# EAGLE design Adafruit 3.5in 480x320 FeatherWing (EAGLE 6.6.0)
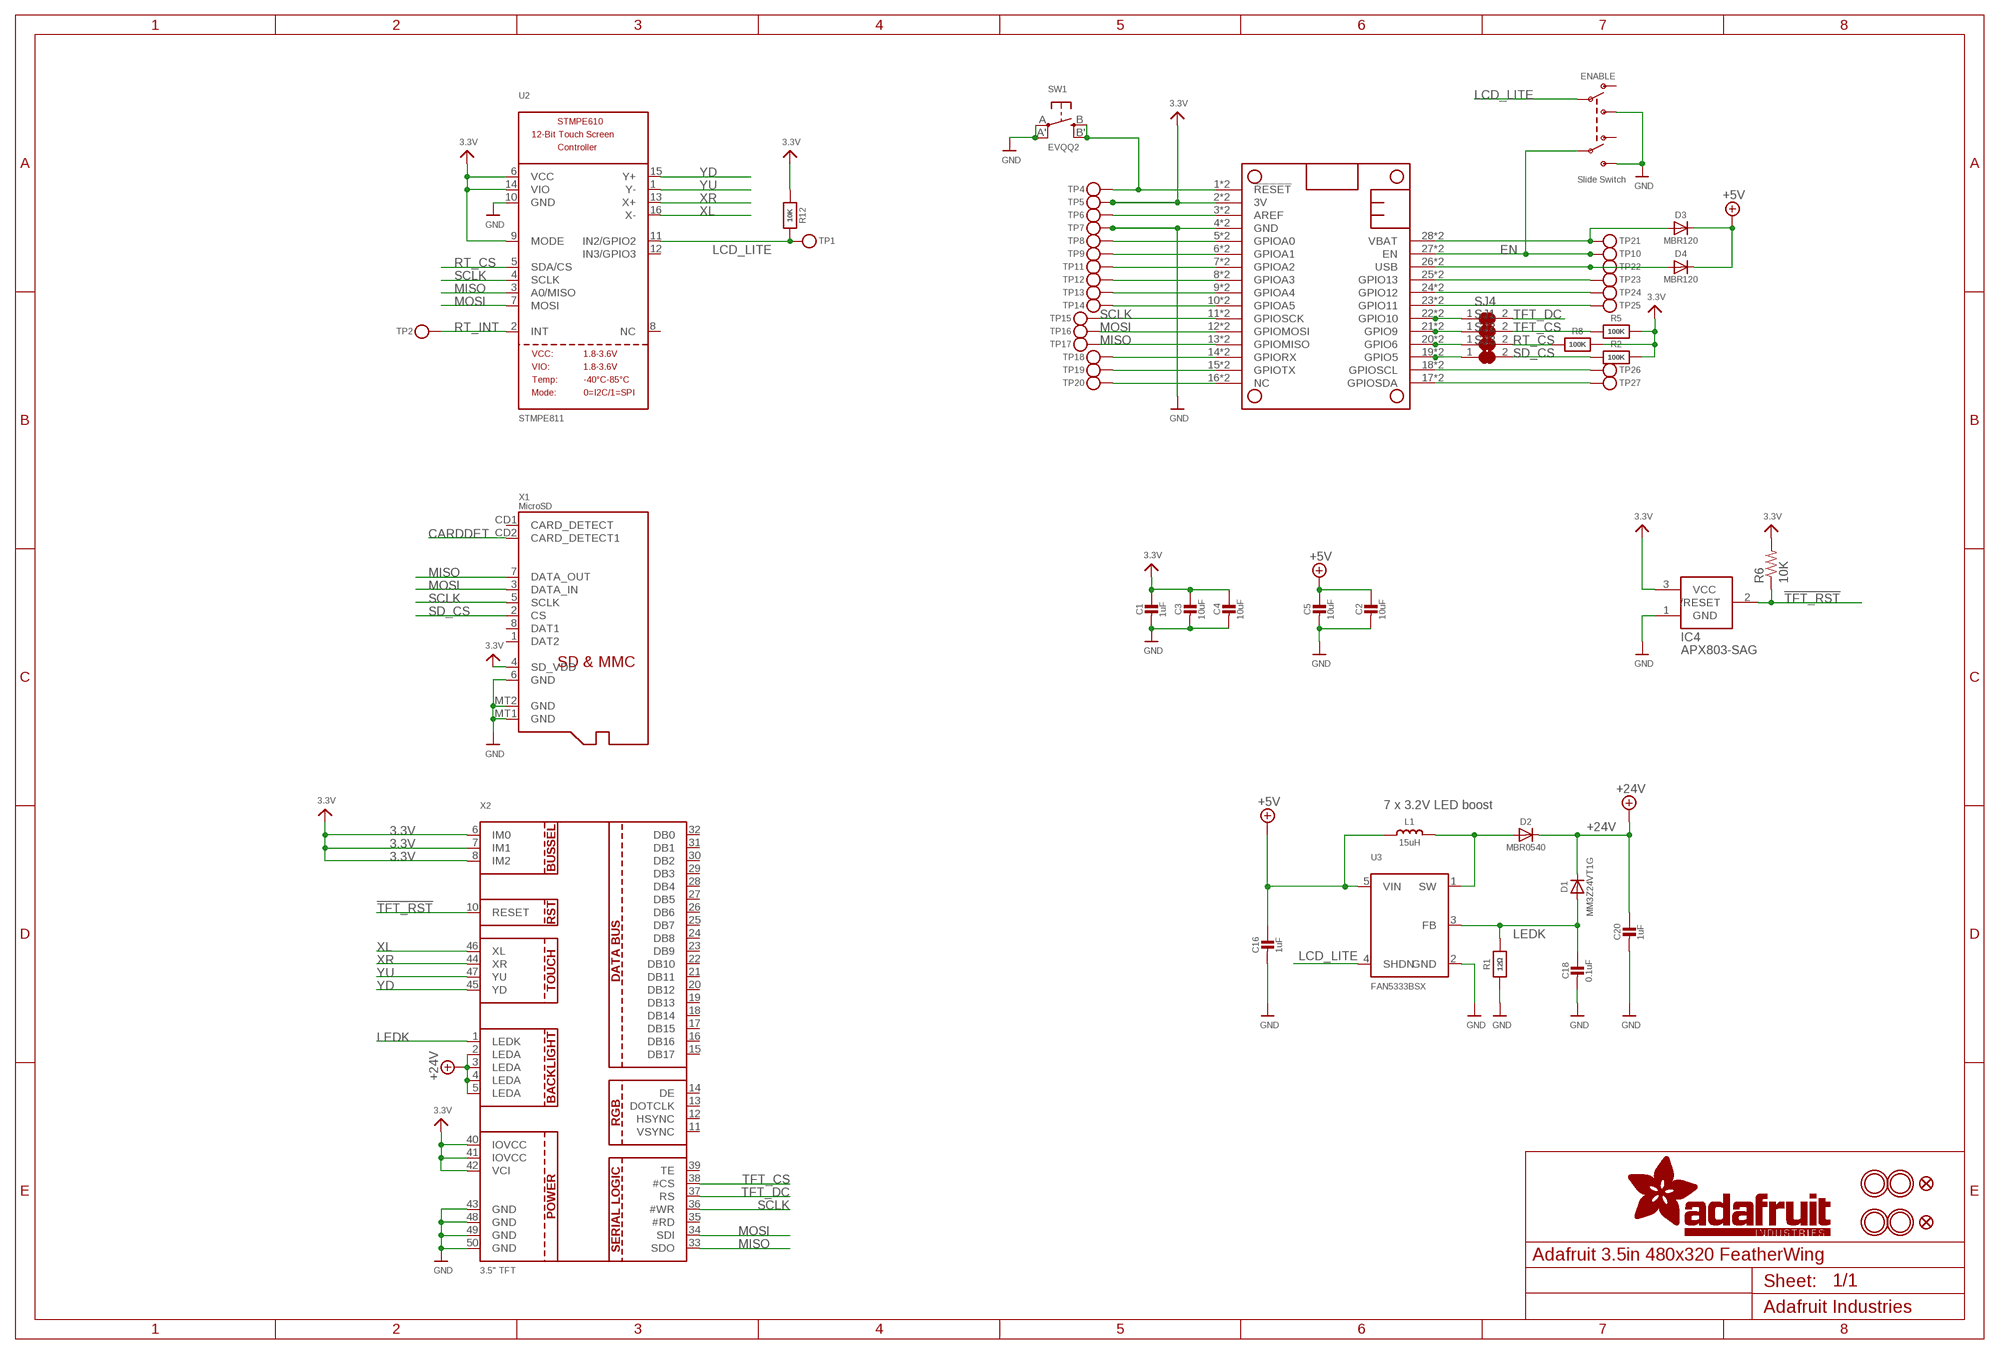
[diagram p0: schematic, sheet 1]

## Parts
C1  1uF  CAP_CERAMIC0805-NOOUTLINE  [0805-NO]
C2  10uF  CAP_CERAMIC0805-NOOUTLINE  [0805-NO]
C3  10uF  CAP_CERAMIC0805-NOOUTLINE  [0805-NO]
C4  10uF  CAP_CERAMIC0805-NOOUTLINE  [0805-NO]
C5  10uF  CAP_CERAMIC0805-NOOUTLINE  [0805-NO]
C16  1uF  CAP_CERAMIC0805-NOOUTLINE  [0805-NO]
C18  0.1uF  CAP_CERAMIC0805-NOOUTLINE  [0805-NO]
C20  1uF  CAP_CERAMIC0805-NOOUTLINE  [0805-NO]
D1  MM3Z24VT1G  DIODESMA  [SMADIODE]
D2  MBR0540  DIODESOD-123  [SOD-123]
D3  MBR120  DIODESOD-123  [SOD-123]
D4  MBR120  DIODESOD-123  [SOD-123]
ENABLE  Slide Switch  SWITCH_DPDTEG1390  [EG1390]
IC4  APX803-SAG  AXP083-SAG  [SOT23]
L1  15uH  INDUCTORNR5040  [INDUCTOR_5X5MM_NR5040_NOTHERMALS]
MS2  FEATHERWING_SMTDUAL  [FEATHERWING_SMT2]
R1  12Ω  RESISTOR0805_NOOUTLINE  [0805-NO]
R2  100K  RESISTOR0805_NOOUTLINE  [0805-NO]
R5  100K  RESISTOR0805_NOOUTLINE  [0805-NO]
R6  10K  R-US_R0805  [R0805]
R8  100K  RESISTOR0805_NOOUTLINE  [0805-NO]
R12  10K  RESISTOR0805_NOOUTLINE  [0805-NO]
SJ1  SOLDERJUMPER_CLOSED  [SOLDERJUMPER_CLOSEDWIRE]
SJ2  SOLDERJUMPER_CLOSED  [SOLDERJUMPER_CLOSEDWIRE]
SJ3  SOLDERJUMPER_CLOSED  [SOLDERJUMPER_CLOSEDWIRE]
SJ4  SOLDERJUMPER_CLOSED  [SOLDERJUMPER_CLOSEDWIRE]
SW1  EVQQ2  SWITCH_TACT_SMT_EVQQ2_SMALL  [EVQ-Q2_SMALLER]
TP1  TESTPOINTPAD2MM  [TESTPOINT_PAD_2MM]
TP2  TESTPOINTPAD2MM  [TESTPOINT_PAD_2MM]
TP4  TESTPOINTPAD2MM  [TESTPOINT_PAD_2MM]
TP5  TESTPOINTPAD2MM  [TESTPOINT_PAD_2MM]
TP6  TESTPOINTPAD2MM  [TESTPOINT_PAD_2MM]
TP7  TESTPOINTPAD2MM  [TESTPOINT_PAD_2MM]
TP8  TESTPOINTPAD2MM  [TESTPOINT_PAD_2MM]
TP9  TESTPOINTPAD2MM  [TESTPOINT_PAD_2MM]
TP10  TESTPOINTPAD2MM  [TESTPOINT_PAD_2MM]
TP11  TESTPOINTPAD2MM  [TESTPOINT_PAD_2MM]
TP12  TESTPOINTPAD2MM  [TESTPOINT_PAD_2MM]
TP13  TESTPOINTPAD2MM  [TESTPOINT_PAD_2MM]
TP14  TESTPOINTPAD2MM  [TESTPOINT_PAD_2MM]
TP15  TESTPOINTPAD2MM  [TESTPOINT_PAD_2MM]
TP16  TESTPOINTPAD2MM  [TESTPOINT_PAD_2MM]
TP17  TESTPOINTPAD2MM  [TESTPOINT_PAD_2MM]
TP18  TESTPOINTPAD2MM  [TESTPOINT_PAD_2MM]
TP19  TESTPOINTPAD2MM  [TESTPOINT_PAD_2MM]
TP20  TESTPOINTPAD2MM  [TESTPOINT_PAD_2MM]
TP21  TESTPOINTPAD2MM  [TESTPOINT_PAD_2MM]
TP22  TESTPOINTPAD2MM  [TESTPOINT_PAD_2MM]
TP23  TESTPOINTPAD2MM  [TESTPOINT_PAD_2MM]
TP24  TESTPOINTPAD2MM  [TESTPOINT_PAD_2MM]
TP25  TESTPOINTPAD2MM  [TESTPOINT_PAD_2MM]
TP26  TESTPOINTPAD2MM  [TESTPOINT_PAD_2MM]
TP27  TESTPOINTPAD2MM  [TESTPOINT_PAD_2MM]
U2  STMPE811  STMPE610  [QFN16_3MM]
U3  FAN5333BSX  FAN5331  [SOT23-5@1]
U$7  MOUNTINGHOLE3.0THIN  [MOUNTINGHOLE_3.0_PLATEDTHIN]
U$9  FIDUCIAL_1MM  [FIDUCIAL_1MM]
U$15  MOUNTINGHOLE3.0THIN  [MOUNTINGHOLE_3.0_PLATEDTHIN]
U$16  MOUNTINGHOLE3.0THIN  [MOUNTINGHOLE_3.0_PLATEDTHIN]
U$17  MOUNTINGHOLE3.0THIN  [MOUNTINGHOLE_3.0_PLATEDTHIN]
U$23  FIDUCIAL_1MM  [FIDUCIAL_1MM]
X1  MicroSD  MICROSD  [MICROSD]
X2  3.5" TFT  DISP_LCD_3.5IN_320X480_50PIN  [TFT_3.5IN_320X480_50PIN]

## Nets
3.3V: C1.1 C3.1 C4.1 IC4.3(VCC) MS2.2'(3V) MS2.2(3V) R2.2 R5.2 R6.2 R8.2 R12.1 TP5.P$1 U2.6(VCC) U2.9(MODE) U2.14(VIO) X1.4(SD_VDD) X2.6(IM0) X2.7(IM1) X2.8(IM2) X2.40(IOVCC) X2.41(IOVCC) X2.42(VCI)
!RESET: MS2.1'(!RESET) MS2.1(!RESET) SW1.B'(S1) SW1.B(S) TP4.P$1
!TFT_RST: IC4.2(/RESET) R6.1 X2.10(RESET)
+5V: C2.1 C5.1 C16.1 D3.C D4.C L1.P$1 U3.5(VIN)
+24V: C20.1 D1.C D2.C X2.2(LEDA) X2.3(LEDA) X2.4(LEDA) X2.5(LEDA)
A: MS2.5'(GPIOA0) MS2.5(GPIOA0) TP8.P$1
AREF: MS2.3'(AREF) MS2.3(AREF) TP6.P$1
B: MS2.6'(GPIOA1) MS2.6(GPIOA1) TP9.P$1
C: MS2.7'(GPIOA2) MS2.7(GPIOA2) TP11.P$1
CARDDET: X1.CD2(CARD_DETECT1)
D: MS2.8'(GPIOA3) MS2.8(GPIOA3) TP12.P$1
E: MS2.9'(GPIOA4) MS2.9(GPIOA4) TP13.P$1
EN: ENABLE.P2 MS2.27'(EN) MS2.27(EN) TP10.P$1
F: MS2.10'(GPIOA5) MS2.10(GPIOA5) TP14.P$1
G: MS2.16'(NC) MS2.16(NC) TP20.P$1
GND: C1.2 C2.2 C3.2 C4.2 C5.2 C16.2 C18.2 C20.2 ENABLE.S1 ENABLE.S2 IC4.1(GND) MS2.4'(GND) MS2.4(GND) R1.1 SW1.A'(P1) SW1.A(P) TP7.P$1 U2.10(GND) U3.2(GND) X1.6(GND) X1.MT1(GND) X1.MT2(GND) X2.43(GND) X2.48(GND) X2.49(GND) X2.50(GND)
H: MS2.19'(GPIO5) MS2.19(GPIO5) SJ3.1
I: MS2.20'(GPIO6) MS2.20(GPIO6) SJ2.1
J: MS2.21'(GPIO9) MS2.21(GPIO9) SJ1.1
K: MS2.22'(GPIO10) MS2.22(GPIO10) SJ4.1
L: MS2.23'(GPIO11) MS2.23(GPIO11) TP25.P$1
LCD_LITE: ENABLE.P1 R12.2 TP1.P$1 U2.11(IN2/GPIO2) U3.4(SHDN)
LEDK: C18.1 D1.A R1.2 U3.3(FB) X2.1(LEDK)
M: MS2.24'(GPIO12) MS2.24(GPIO12) TP24.P$1
MISO: MS2.13'(GPIOMISO) MS2.13(GPIOMISO) TP17.P$1 U2.3(A0/MISO) X1.7(DATA_OUT) X2.33(SDO)
MOSI: MS2.12'(GPIOMOSI) MS2.12(GPIOMOSI) TP16.P$1 U2.7(MOSI) X1.3(DATA_IN) X2.34(SDI)
N: MS2.25'(GPIO13) MS2.25(GPIO13) TP23.P$1
N$3: D2.A L1.P$2 U3.1(SW)
RT_CS: R8.1 SJ2.2 U2.5(SDA/CS)
RT_INT: TP2.P$1 U2.2(INT)
RX: MS2.14'(GPIORX) MS2.14(GPIORX) TP18.P$1
SCL: MS2.18'(GPIOSCL) MS2.18(GPIOSCL) TP26.P$1
SCLK: MS2.11'(GPIOSCK) MS2.11(GPIOSCK) TP15.P$1 U2.4(SCLK) X1.5(SCLK) X2.36(#WR)
SD_CS: R2.1 SJ3.2 X1.2(CS)
SDA: MS2.17'(GPIOSDA) MS2.17(GPIOSDA) TP27.P$1
TFT_CS: R5.1 SJ1.2 X2.38(#CS)
TFT_DC: SJ4.2 X2.37(RS)
TX: MS2.15'(GPIOTX) MS2.15(GPIOTX) TP19.P$1
USB: D4.A MS2.26'(USB) MS2.26(USB) TP22.P$1
VBAT: D3.A MS2.28'(VBAT) MS2.28(VBAT) TP21.P$1
XL: U2.16(X-) X2.46(XL)
XR: U2.13(X+) X2.44(XR)
YD: U2.15(Y+) X2.45(YD)
YU: U2.1(Y-) X2.47(YU)
Unconnected: ENABLE.O1 ENABLE.O2 U2.8(NC) U2.12(IN3/GPIO3) X1.1(DAT2) X1.8(DAT1) X1.CD1(CARD_DETECT) X2.11(VSYNC) X2.12(HSYNC) X2.13(DOTCLK) X2.14(DE) X2.15(DB17) X2.16(DB16) X2.17(DB15) X2.18(DB14) X2.19(DB13) X2.20(DB12) X2.21(DB11) X2.22(DB10) X2.23(DB9) X2.24(DB8) X2.25(DB7) X2.26(DB6) X2.27(DB5) X2.28(DB4) X2.29(DB3) X2.30(DB2) X2.31(DB1) X2.32(DB0) X2.35(#RD) X2.39(TE)

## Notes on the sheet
- 7 x 3.2V LED boost

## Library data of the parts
C1-C5 C16 C18 C20 = microbuilder:CAP_CERAMIC: Ceramic Capacitors
D1-D4 = microbuilder:DIODE: Diode
ENABLE = microbuilder:SWITCH_DPDT: Switch - DPDT A DPDT Switch acts like an SPDT switch, but has a pair of switches instead of just one. Vertical - 0.3A @ 6V SMT - Digikey: JS202011SCQN
IC4 = adafruit:AXP083
L1 = microbuilder:INDUCTOR: Inductors
MS2 = microbuilder:FEATHERWING
R1 R2 R5 R8 R12 = microbuilder:RESISTOR: Resistors
R6 = rcl:R-US_: RESISTOR, American symbol
SJ1-SJ4 = microbuilder:SOLDERJUMPER_CLOSED: Solder Jumper - Closed
SW1 = microbuilder:SWITCH_TACT_SMT: SMT Tact Switches 6x6mm - Digikey: P12940SCT-ND KMR2 (4.6x2.8mm) - Digikey: 401-1426-1-ND EVQ-PQHB55 - Light Touch, 160GF (4.5x4.5mm) - Digikey: P8090SCT-ND KMT0 - KMT021 NGJ LHS (etc.) IP68/Waterproof - Digikey: CKN10289CT-ND
TP1 TP2 TP4-TP27 = microbuilder:TESTPOINT: Test Point
U2 = microbuilder:STMPE610: STMPE610 - 12-Bit Touch Screen Controller
U3 = microbuilder:FAN5331: FAN5331 - LED/OLED 20V Boost Converter Digikey: FAN5331SXCT-ND
U$7 U$15-U$17 = microbuilder:MOUNTINGHOLE: Mounting Hole; BOM: EXCLUDE
U$9 U$23 = microbuilder:FIDUCIAL: Fiducial Alignment Points; BOM: EXCLUDE
X1 = microbuilder:MICROSD: MicroSD/Transflash Card Holder with SPI pinout 3M: 2908-05WB-MG 4UConnector: 19656 Footprint courtesy: Adafruit Industries
X2 = microbuilder:DISP_LCD_3.5IN_320X480_50PIN: DT350HV15-T - 3.5" 320x480 TFT Display, 50 Pin Connector

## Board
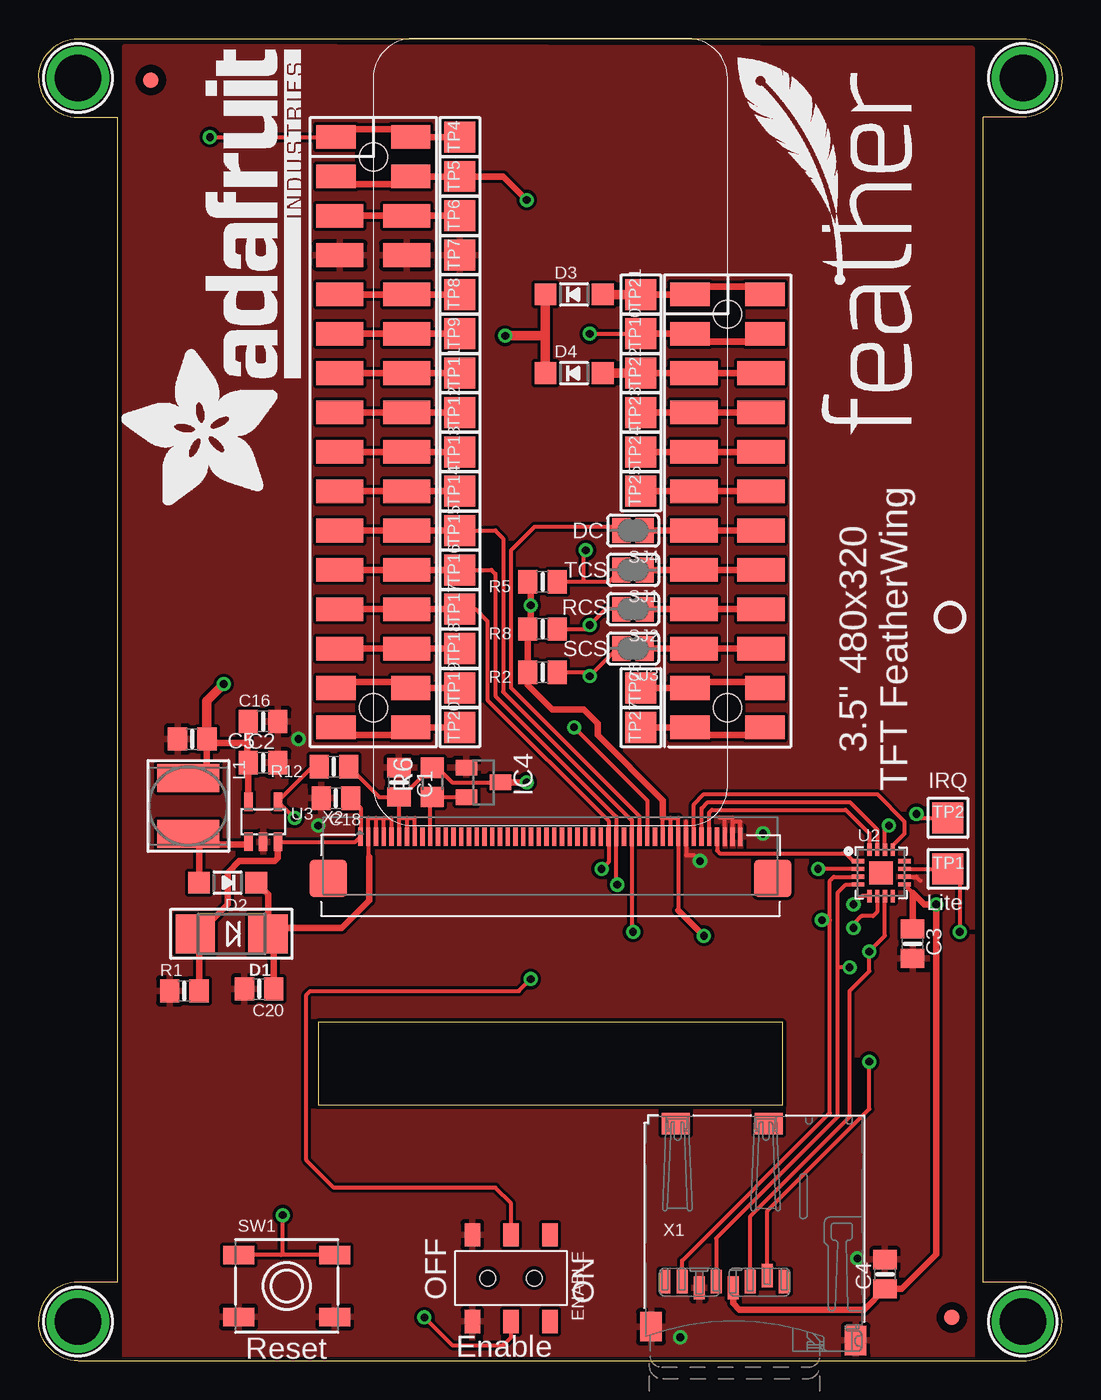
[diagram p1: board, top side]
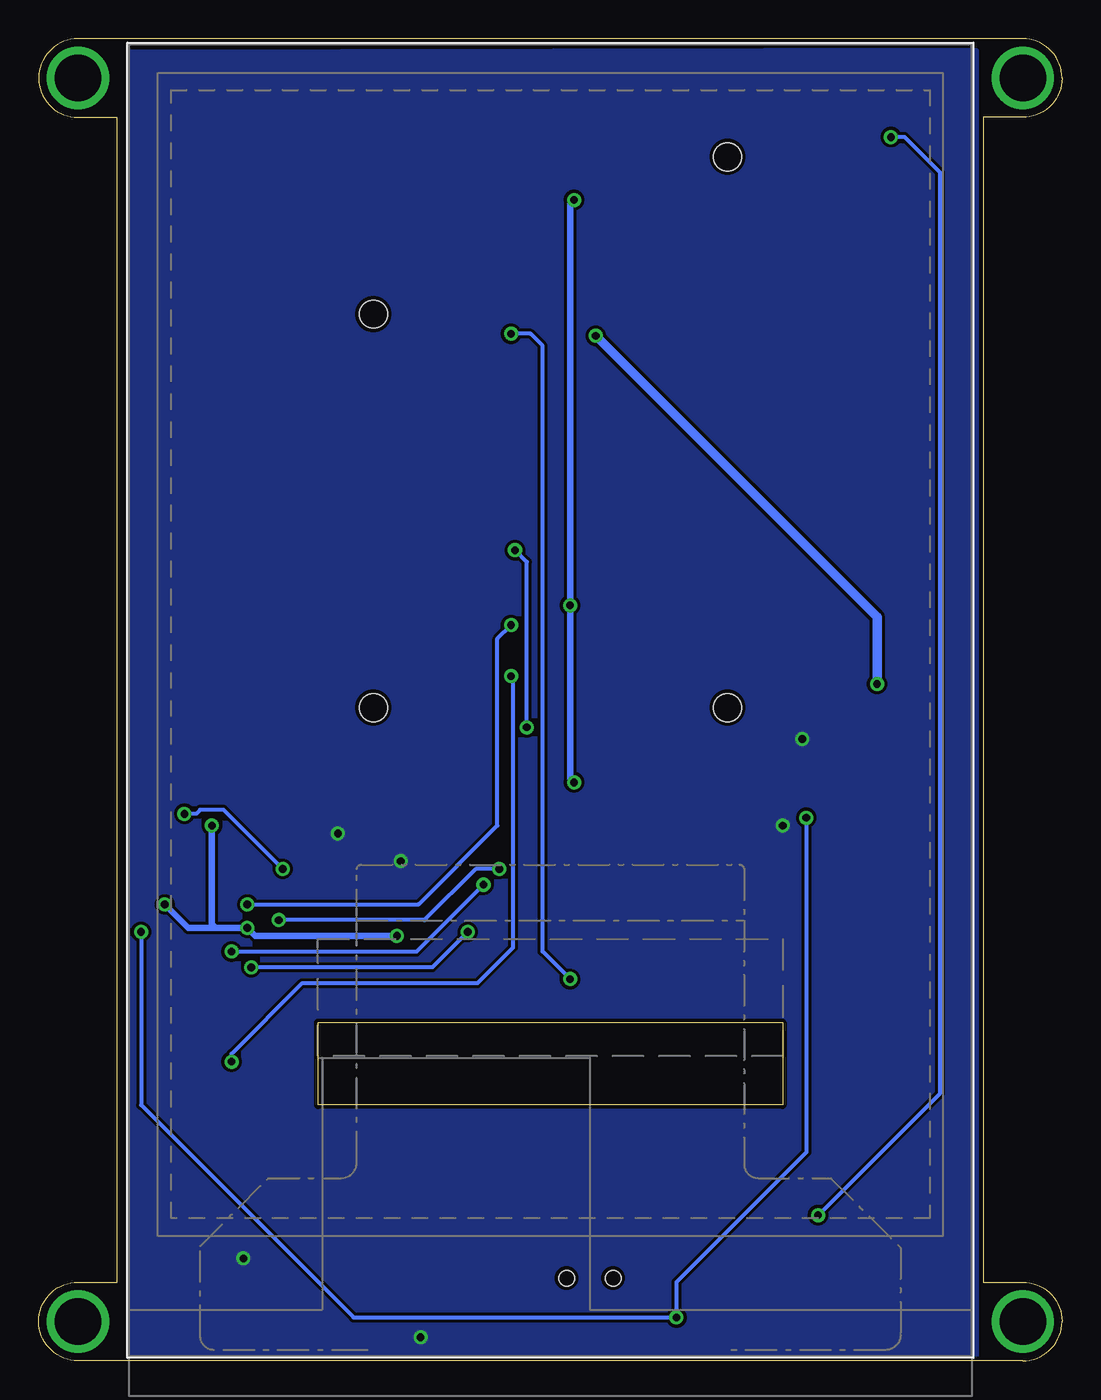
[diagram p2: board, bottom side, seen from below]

Size 66.04 x 85.34 mm. Coordinates in mm from the lower left corner, seen from the top.
Outline: 2.54,0 63.5,0 arc90 66.04,2.54 arc90 63.5,5.08 60.96,5.08 60.96,80.26 63.5,80.26 arc90 66.04,82.8 arc90 63.5,85.34 2.54,85.34 arc90 0,82.8 arc90 2.54,80.26 5.08,80.26 5.08,5.08 2.54,5.08 arc90 0,2.54 arc90 2.54,0
Outline: 18.03,21.84 18.03,16.51 48.01,16.51 48.01,21.84 18.03,21.84
Copper layers (1*16): Top 0.035mm / dielectric 1.5mm / Bottom 0.035mm
Design rules "adafruit *": minimum track width 8mil, minimum drill 15.5mil, track to track 8mil, track to pad 8mil, pad to pad 8mil, via to via 8mil, smd to smd 8mil, copper to edge 10mil, drill to drill 8mil, minimum pad ring 10mil, minimum via ring 8mil, stop-mask expansion 2mil, vias tented up to drill 20mil, thermal gap 10mil
tRestrict: area 44.5,33.7 to 44.6,34; area 45,33.7 to 45.1,34

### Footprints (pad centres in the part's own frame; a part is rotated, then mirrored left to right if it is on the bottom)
0805-NO = smd 1.24 x 1.5: 1 -0.95,0; 2 0.95,0
SMADIODE = smd 2.54 x 2.54: A 2.349,0; C -2.349,0
SOD-123 = smd 1.4 x 1.4: A 1.85,0; C -1.85,0
EG1390 = smd 1 x 1.5: O1 -2.5,2.8; O2 -2.5,-2.8; P1 0,2.8; P2 0,-2.8; S1 2.5,2.8; S2 2.5,-2.8 | hole 1: 1.5,0; -1.5,0
SOT23 = smd 1 x 1.4: 1 -0.95,-1.1; 2 0.95,-1.1; 3 0,1.1
INDUCTOR_5X5MM_NR5040_NOTHERMALS = smd 1.8 x 4: P$1 -1.8,0; P$2 1.8,0
FEATHERWING_SMT2 = smd 1.524 x 2.54: 1 6.35,2.413; 1' 6.35,-2.413; 2 8.89,2.413; 2' 8.89,-2.413; 15 41.91,2.413; 15' 41.91,-2.413; 16 44.45,2.413; 16' 44.45,-2.413; 17 44.45,20.447; 17' 44.45,25.273; 18 41.91,20.447; 18' 41.91,25.273; 27 19.05,20.447; 27' 19.05,25.273; 28 16.51,20.447; 28' 16.51,25.273 | smd 1.524 x 3.048: 3 11.43,2.159; 3' 11.43,-2.159; 4 13.97,2.159; 4' 13.97,-2.159; 5 16.51,2.159; 5' 16.51,-2.159; 6 19.05,2.159; 6' 19.05,-2.159; 7 21.59,2.159; 7' 21.59,-2.159; 8 24.13,2.159; 8' 24.13,-2.159; 9 26.67,2.159; 9' 26.67,-2.159; 10 29.21,2.159; 10' 29.21,-2.159; 11 31.75,2.159; 11' 31.75,-2.159; 12 34.29,2.159; 12' 34.29,-2.159; 13 36.83,2.159; 13' 36.83,-2.159; 14 39.37,2.159; 14' 39.37,-2.159; 19 39.37,20.701; 19' 39.37,25.019; 20 36.83,20.701; 20' 36.83,25.019; 21 34.29,20.701; 21' 34.29,25.019; 22 31.75,20.701; 22' 31.75,25.019; 23 29.21,20.701; 23' 29.21,25.019; 24 26.67,20.701; 24' 26.67,25.019; 25 24.13,20.701; 25' 24.13,25.019; 26 21.59,20.701; 26' 21.59,25.019 | hole 1.8: 17.78,22.86; 43.18,22.86; 7.62,0; 43.18,0
R0805 = smd 1.3 x 1.5: 1 -0.95,0; 2 0.95,0
SOLDERJUMPER_CLOSEDWIRE = smd 1.168 x 1.6: 1 -0.762,0; 2 0.762,0 | smd 0.635 x 0.203: WIRE 0,0
EVQ-Q2_SMALLER = smd 2 x 1.2: A -3.1,-2; A' 3.1,-2; B -3.1,2; B' 3.1,2
TESTPOINT_PAD_2MM = smd 2 x 2: P$1 0,0
QFN16_3MM = smd 0.8 x 0.28: 1 -1.5,0.75; 2 -1.5,0.25; 3 -1.5,-0.25; 4 -1.5,-0.75; 9 1.5,-0.75; 10 1.5,-0.25; 11 1.5,0.25; 12 1.5,0.75 | smd 0.28 x 0.8: 5 -0.75,-1.5; 6 -0.25,-1.5; 7 0.25,-1.5; 8 0.75,-1.5; 13 0.75,1.5; 14 0.25,1.5; 15 -0.25,1.5; 16 -0.75,1.5 | smd 1.5 x 1.5: THERMAL 0,0
SOT23-5@1 = smd 0.55 x 1.2: 1 -0.95,-1.3; 2 0,-1.3; 3 0.95,-1.3; 4 0.95,1.3; 5 -0.95,1.3
MOUNTINGHOLE_3.0_PLATEDTHIN = drill 3 pad 3.6: P$1 0,0
FIDUCIAL_1MM = smd 1 x 1: 1 0,0
MICROSD = smd 0.7 x 1.5: 1 9,-10.64; 2 7.9,-10.24; 3 6.8,-10.64; 4 5.7,-11.04; 5 4.6,-10.64; 6 3.5,-11.04; 7 2.4,-10.64; 8 1.3,-10.64 | smd 1.8 x 1.4: CD1 2,-0.44; CD2 8,-0.44 | smd 1.4 x 1.9: MT1 0.4,-13.54; MT2 13.6,-14.44
TFT_3.5IN_320X480_50PIN = smd 0.275 x 1.2 bottom: 1 12.25,-3.76; 2 11.75,-3.76; 3 11.25,-3.76; 4 10.75,-3.76; 5 10.25,-3.76; 6 9.75,-3.76; 7 9.25,-3.76; 8 8.75,-3.76; 9 8.25,-3.76; 10 7.75,-3.76; 11 7.25,-3.76; 12 6.75,-3.76; 13 6.25,-3.76; 14 5.75,-3.76; 15 5.25,-3.76; 16 4.75,-3.76; 17 4.25,-3.76; 18 3.75,-3.76; 19 3.25,-3.76; 20 2.75,-3.76; 21 2.25,-3.76; 22 1.75,-3.76; 23 1.25,-3.76; 24 0.75,-3.76; 25 0.25,-3.76; 26 -0.25,-3.76; 27 -0.75,-3.76; 28 -1.25,-3.76; 29 -1.75,-3.76; 30 -2.25,-3.76; 31 -2.75,-3.76; 32 -3.25,-3.76; 33 -3.75,-3.76; 34 -4.25,-3.76; 35 -4.75,-3.76; 36 -5.25,-3.76; 37 -5.75,-3.76; 38 -6.25,-3.76; 39 -6.75,-3.76; 40 -7.25,-3.76; 41 -7.75,-3.76; 42 -8.25,-3.76; 43 -8.75,-3.76; 44 -9.25,-3.76; 45 -9.75,-3.76; 46 -10.25,-3.76; 47 -10.75,-3.76; 48 -11.25,-3.76; 49 -11.75,-3.76; 50 -12.25,-3.76 | smd 2.4 x 2.4 bottom: PAD1 14.35,-6.46; PAD2 -14.35,-6.46

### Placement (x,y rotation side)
C1  23.24,37.34 90 top
C2  14.48,38.61 0 top
C3  56.39,26.92 270 top
C4  54.61,5.59 90 top
C5  9.91,40.13 180 top
C16  14.48,41.27 0 top
C18  19.18,36.32 180 top
C20  14.22,24 180 top
D1  12.45,27.56 180 top
D2  12.19,30.86 180 top
D3  34.54,68.83 0 top
D4  34.54,63.75 0 top
ENABLE  30.48,5.33 180 top
IC4  28.7,37.34 270 top
L1  9.65,35.81 270 top
MS2  21.59,85.34 270 top
R1  9.4,23.88 0 top
R2  32.51,44.45 180 top
R5  32.51,50.29 180 top
R6  25.4,37.34 90 top
R8  32.51,47.24 180 top
R12  19.05,38.35 180 top
SJ1  38.35,51.05 180 top
SJ2  38.35,48.51 180 top
SJ3  38.35,45.97 180 top
SJ4  38.35,53.59 180 top
SW1  16,4.83 0 top
TP1  58.67,31.75 0 top
TP2  58.67,35.05 0 top
TP4  27.18,78.99 90 top
TP5  27.18,76.45 90 top
TP6  27.18,73.91 90 top
TP7  27.18,71.37 90 top
TP8  27.18,68.83 90 top
TP9  27.18,66.29 90 top
TP10  38.86,66.29 90 top
TP11  27.18,63.75 90 top
TP12  27.18,61.21 90 top
TP13  27.18,58.67 90 top
TP14  27.18,56.13 90 top
TP15  27.18,53.59 90 top
TP16  27.18,51.05 90 top
TP17  27.18,48.51 90 top
TP18  27.18,45.97 90 top
TP19  27.18,43.43 90 top
TP20  27.18,40.89 90 top
TP21  38.86,68.83 90 top
TP22  38.86,63.75 90 top
TP23  38.86,61.21 90 top
TP24  38.86,58.67 90 top
TP25  38.86,56.13 90 top
TP26  38.86,43.43 90 top
TP27  38.86,40.89 90 top
U2  54.36,31.5 0 top
U3  14.48,34.8 0 top
U$7  2.54,2.54 0 top
U$9  58.93,2.79 0 top
U$11  [FEATHERLOGO]  56.39,59.82 90 top
U$15  63.5,2.54 0 top
U$16  2.54,82.8 0 top
U$17  63.5,82.8 0 top
U$19  [ADAFRUIT_TEXT_30MM]  16.89,54.99 90 top
U$23  7.24,82.68 0 top
U$37  [PCBFEAT-REV-040]  58.8,48.01 90 top
X1  39.12,15.75 0 top
X2  33.02,37.59 0 bottom

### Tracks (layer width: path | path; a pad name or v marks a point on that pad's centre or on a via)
3.3V  (via drill 0.5)
  Top 0.254: X2.6 23.27,35.05 | 23.27,35.05 23.77,35.05 | 23.77,35.05 24.27,35.05 X2.8 | X2.7 23.77,35.05 | 23.27,35.05 23.27,36.39 C1.1 | C1.1 23.43,36.39 24.89,37.85 24.96,37.85 R6.2 25.72,38.29 26.67,37.34 IC4.3 | U2.9 56.39,30.21 | U2.6 54.11,28.96 53.85,28.7 53.09,28.7 52.58,28.19 v52.58,27.94 | X2.40 40.27,35.05 40.77,35.05 | 40.77,35.05 41.27,35.05 X2.42 41.27,29.09 | X2.41 40.77,35.05 | R12.1 21.97,36.39 C1.1 | U2.14 54.61,34.29 v54.86,34.54
  Top 0.406: IC4.3 v31.5,37.34 | X1.4 44.82,3.7 45.21,3.3 53.27,3.3 C4.1 55.69,4.64 57.91,6.86 v57.91,29.46 57.14,29.46 56.39,30.21 C3.1 | v31.5,74.93 29.97,76.45 TP5.P$1 MS2.2 23.88,76.45 23.37,75.95 19.69,75.95 MS2.2' | 41.27,29.09 v42.93,27.43 | 40.27,35.05 40.27,36.18 36.07,40.39 36.07,41.15 35.18,42.04 33.15,42.04 31.56,43.62 R2.2 R8.2 31.75,47.43 v31.75,48.77 31.75,50.1 R5.2
  Bottom 0.254: v31.5,37.34 31.75,37.59 | 31.75,48.01 v31.75,48.77
  Bottom 0.406: 54.61,27.94 v52.58,27.94 52.07,27.43 v42.93,27.43 | 54.61,27.94 56.39,27.94 v57.91,29.46 | 31.75,37.59 31.75,48.01 31.75,74.68 v31.5,74.93 | v54.86,34.54 54.86,28.19 54.61,27.94
!RESET  (via drill 0.5)
  Top 0.254: SW1.B' 15.62,6.83 | 15.62,6.83 SW1.B | 15.62,6.83 15.75,6.96 v15.75,9.4 | v11.05,78.99 MS2.1'
  Top 0.406: TP4.P$1 MS2.1 23.75,78.99 23.24,79.5 19.69,79.5 MS2.1'
  Bottom 0.254: v15.75,9.4 7.87,17.27 7.87,76.71 10.16,78.99 v11.05,78.99
!TFT_RST
  Top 0.254: X2.10 25.27,36.26 R6.1 IC4.2
+5V  (via drill 0.5)
  Top 0.406: 13.46,39.88 13.46,38.61 C2.1 U3.5 | L1.P$1 10.86,37.61 C5.1 10.86,39.88 13.46,39.88 | 13.46,39.88 13.46,41.21 C16.1
  Top 0.61: D4.C 32.69,66.17 | 32.69,66.17 D3.C | 32.69,66.17 v30.1,66.17 | v11.94,43.69 10.86,42.61 C5.1
  Bottom 0.61: v30.1,66.17 11.94,48.01 v11.94,43.69
+24V
  Top 0.254: 21.77,35.05 21.27,35.05 X2.2 21.27,32.58 21.34,32.51 | 21.77,35.05 22.27,35.05 | 22.27,35.05 22.77,35.05 X2.5 | X2.4 22.27,35.05 | X2.3 21.77,35.05
  Top 0.406: D2.C 14.8,30.11 D1.C | D1.C 15.17,27.18 C20.1 | 21.34,32.51 21.34,29.72 19.56,27.94 15.18,27.94 D1.C
A
  Top 0.406: TP8.P$1 MS2.5 MS2.5'
AREF
  Top 0.406: MS2.3' MS2.3 TP6.P$1
B
  Top 0.406: MS2.6' MS2.6 TP9.P$1
C
  Top 0.406: TP11.P$1 MS2.7 MS2.7'
D
  Top 0.406: MS2.8' MS2.8 TP12.P$1
E
  Top 0.406: TP13.P$1 MS2.9 MS2.9'
EN  (via drill 0.5)
  Top 0.254: ENABLE.P2 30.48,10.16 29.46,11.18 19.05,11.18 17.27,12.95 17.27,23.62 17.53,23.88 30.99,23.88 v31.75,24.64 | v35.56,66.29 TP10.P$1
  Top 0.406: TP10.P$1 MS2.27 42.55,65.79 46.48,65.79 46.86,66.17 MS2.27'
  Bottom 0.254: v31.75,24.64 33.53,26.42 33.53,65.53 34.29,66.29 v35.56,66.29
F
  Top 0.406: TP14.P$1 MS2.10 MS2.10'
G
  Top 0.406: TP20.P$1 MS2.16 23.75,40.89 23.24,40.39 19.69,40.39 MS2.16'
GND  (via drill 0.5)
  Top 0.254: X2.48 44.27,35.05 | 44.27,35.05 43.94,35.05 | X2.49 44.77,34.8 | 44.77,34.8 44.77,35.05 44.27,35.05 | 41.77,34.8 X2.43 41.77,32.65 42.28,32.65 v42.67,32.26 | X2.50 45.27,34.8 44.77,34.8 | U2.10 56.64,31.25 56.9,30.99
  other vias: 46.74,34.04 18.03,34.54 16.76,40.13 41.4,1.52 52.83,6.6
  pour Top: 5.59,84.84 5.59,0 60.2,-0.13 60.2,84.71
  pour Bottom: 5.59,84.58 5.59,-0.25 60.2,-0.38 60.2,84.45
H
  Top 0.406: SJ3.1 MS2.19 MS2.19'
I
  Top 0.406: MS2.20' MS2.20 SJ2.1
J
  Top 0.406: SJ1.1 MS2.21 MS2.21'
K
  Top 0.406: MS2.22' MS2.22 SJ4.1
L
  Top 0.406: TP25.P$1 41.4,56.13 41.4,56.39 42.29,56.39 MS2.23 MS2.23'
LCD_LITE  (via drill 0.5)
  Top 0.254: U2.11 TP1.P$1 59.44,30.99 v59.44,27.69 | v16.51,35.05 16.47,35.05 U3.4 17.68,38.35 R12.2 | v24.89,2.79 26.67,1.02 29.97,1.02 30.48,1.52 ENABLE.P1
  Bottom 0.254: v16.51,35.05 16.51,13.46 24.89,5.08 v24.89,2.79 45.72,2.79 59.44,16.51 v59.44,27.69
LEDK
  Top 0.254: C18.1 20.77,35.68 X2.1 20.44,33.5 U3.3
  Top 0.406: D1.A 10.29,27.56 | 10.29,27.56 12.19,29.46 12.19,31.5 12.95,32.26 15.24,32.26 15.43,32.45 U3.3 | 10.29,27.56 10.35,27.5 R1.2
M
  Top 0.406: MS2.24' MS2.24 TP24.P$1
MISO  (via drill 0.5)
  Top 0.254: TP17.P$1 28.19,48.51 28.96,47.75 28.96,42.67 36.77,34.86 X2.33 36.77,32.2 v36.32,31.75 | X1.7 41.52,6.46 51.05,16 51.05,28.45 | 51.05,28.45 51.05,30.99 51.31,31.24 U2.3 | v50.55,28.45 51.05,28.45
  Top 0.406: TP17.P$1 MS2.13 MS2.13'
  Bottom 0.254: v36.32,31.75 37.85,31.75 41.15,28.45 v50.55,28.45
MOSI  (via drill 0.5)
  Top 0.254: TP16.P$1 29.21,51.05 29.46,50.8 29.46,42.93 37.27,35.12 X2.34 37.27,30.8 v37.34,30.73 | X1.3 45.92,9.34 52.32,15.75 52.32,23.88 53.59,25.15 v53.59,26.42 54.61,27.43 U2.7
  Top 0.406: TP16.P$1 MS2.12 MS2.12'
  Bottom 0.254: v53.59,26.42 41.66,26.42 v37.34,30.73
N
  Top 0.406: TP23.P$1 MS2.25 MS2.25'
N$3
  Top 0.406: L1.P$2 10.34,33.32 | 10.34,33.32 D2.A | U3.1 13.35,33.32 10.34,33.32
RT_CS  (via drill 0.5)
  Top 0.254: SJ2.2 36.58,48.51 v35.56,47.5 35.31,47.24 R8.1 | U2.5 53.11,30 v52.58,29.46
  Bottom 0.254: v52.58,29.46 41.53,29.46 36.45,34.54 36.45,46.61 v35.56,47.5
RT_INT  (via drill 0.5)
  Top 0.254: U2.2 v50.29,31.75 | v56.64,35.31 56.9,35.05 TP2.P$1
  Bottom 0.254: v50.29,31.75 53.85,35.31 54.1,35.56 55.63,35.56 55.88,35.31 56.39,35.31 v56.64,35.31
RX
  Top 0.406: TP18.P$1 MS2.14 MS2.14'
SCL
  Top 0.406: TP26.P$1 MS2.18 42.42,43.81 46.48,43.81 MS2.18'
SCLK  (via drill 0.5)
  Top 0.254: TP15.P$1 29.46,53.59 29.97,53.09 29.97,43.18 38.27,34.88 X2.36 38.27,27.77 v38.35,27.69 | X1.5 43.72,7.9 51.56,15.75 51.56,25.4 | 51.56,25.4 51.56,30.23 52.08,30.75 U2.4 | v52.32,25.4 51.56,25.4
  Top 0.406: TP15.P$1 MS2.11 MS2.11'
  Bottom 0.254: v38.35,27.69 40.64,25.4 v52.32,25.4
SD_CS  (via drill 0.5)
  Top 0.254: X1.2 47.02,9.68 53.59,16.26 v53.59,19.3 | R2.1 35.31,44.45 v35.56,44.2 37.34,45.97 SJ3.2
  Bottom 0.254: v53.59,19.3 53.59,19.81 49.02,24.38 37.72,24.38 35.43,26.67 35.43,44.07 v35.56,44.2
SDA
  Top 0.406: TP27.P$1 MS2.17 42.55,40.39 46.48,40.39 46.86,40.77 MS2.17'
TFT_CS  (via drill 0.5)
  Top 0.254: v34.54,40.89 39.27,36.17 X2.38 | R5.1 35.18,50.29 | 35.18,50.29 36.83,50.29 SJ1.2 | 35.18,50.29 35.18,52.2 v35.31,52.32
  Bottom 0.254: v34.54,40.89 34.54,51.56 v35.31,52.32
TFT_DC
  Top 0.254: X2.37 38.77,35.14 30.48,43.43 30.48,52.32 32,53.85 37.34,53.85 SJ4.2
TX
  Top 0.406: TP19.P$1 MS2.15 23.75,43.43 23.37,43.81 19.56,43.81 MS2.15'
USB
  Top 0.406: MS2.26' MS2.26 TP22.P$1
  Top 0.61: TP22.P$1 D4.A
VBAT
  Top 0.406: TP21.P$1 MS2.28 42.55,69.34 46.23,69.34 46.74,68.83 MS2.28'
  Top 0.61: D3.A TP21.P$1
XL
  Top 0.254: X2.46 43.27,35.4 43.43,35.56 52.07,35.56 53.59,34.04 53.59,33.01 U2.16
XR
  Top 0.254: X2.44 42.27,35.92 42.93,36.58 54.1,36.58 55.88,34.8 55.88,34.04 55.12,33.27 55.12,33.01 U2.13
YD
  Top 0.254: X2.45 42.77,35.66 43.18,36.07 52.32,36.07 54.1,34.29 U2.15
YU
  Top 0.254: X2.47 43.77,32.94 43.94,32.77 52.07,32.77 52.59,32.25 U2.1

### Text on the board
tPlace: DC | TCS | RCS | 3.5" 480x320 / TFT FeatherWing | SCS | IRQ | Lite | OFF | ON | Reset | Enable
